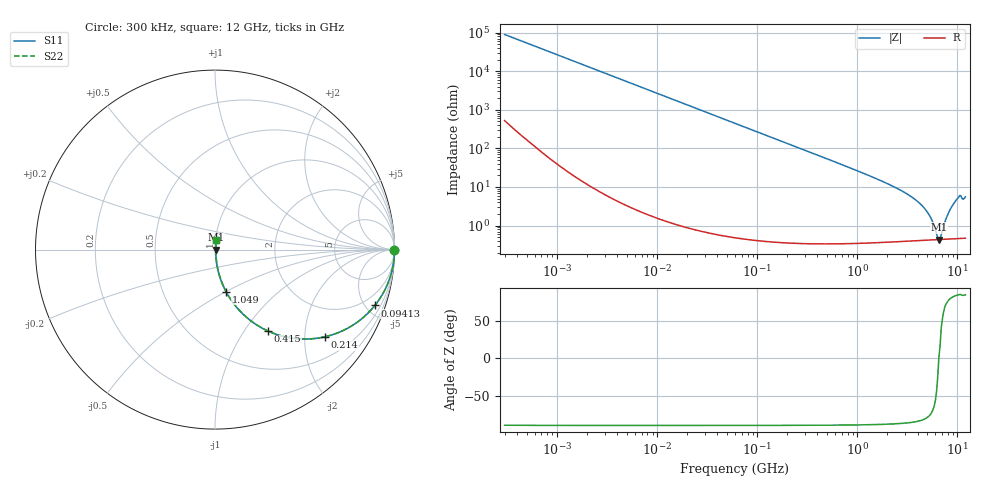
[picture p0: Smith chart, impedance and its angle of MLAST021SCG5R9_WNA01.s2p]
! MLAST021SCG5R9_WNA01  S-PARAMETER MODEL  ( General Type )
! Model Generated by TAIYO YUDEN Corporation (http://www.ty-top.com)
! Version 1.0
! TAIYO YUDEN Control No. 220901
! Copyright(c) 2022 TAIYO YUDEN CO.,LTD. All Rights Reserved.
! Product Description (link to TY-COMPAS)
! https://ds.yuden.co.jp/TYCOMPAS/or/detail?pn=MLAST021SCG5R9CWNA01&u=M
! Products Name : Multilayer Ceramic Capacitors
! Characteristics :
!  Capacitance : 5.9 pF , Rated Voltage : 25V , TCC : CG / C0G
!  Case Size : 0.25 x 0.125 / 0.0098 x 0.0049 [mm/inch] , Thickness : 0.125 / 0.0049 [mm/inch]
!  (Conditions: Temperature = 25 degC , DC Bias Current/Voltage = 0A / 0V)
! External Node Assignments :
!  1  o---| |---o  2
! GND o---------o GND
! Frequency Range : 0.3MHz  -  12000MHz  [ 401 STEP ]
# MHz S RI R 50
! Freq[MHz].  S11 Real  S11 Imag  S21 Real  S21 Imag  S12 Real  S12 Imag  S22 Real  S22 Imag
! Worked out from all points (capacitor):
!   401 points, 300 kHz to 12 GHz, reference 50 ohm
!   read as one part in series: C = 5.9 pF near 316.3 kHz
!   lowest |Z| = 436 mohm at 6.525 GHz (marker M1)
!   series resonance near 6.515 GHz, so ESL is about 100 pH
!   S11 on the Smith chart (normalised r, x): 300 kHz: open; 94.13 MHz: 1.01, -5.73; 214 MHz: 1.01, -2.52; 415 MHz: 1.01, -1.29; 1.049 GHz: 1.01, -0.50; 12 GHz: 1.01, +0.11
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0.3  1 -0.00111  7.74e-06 0.00111  7.74e-06 0.00111  1 -0.00111
1.769972  1 -0.00656  4.92e-05 0.00656  4.92e-05 0.00656  1 -0.00656
10.44266  0.9985 -0.0387  0.00152 0.0387  0.00152 0.0387  0.9985 -0.0387
27.82928  0.9894 -0.1021  0.0106 0.1021  0.0106 0.1021  0.9894 -0.1021
60  0.9526 -0.2119  0.0474 0.2119  0.0474 0.2119  0.9526 -0.2119
94.13233  0.8911 -0.3108  0.1089 0.3108  0.1089 0.3108  0.8911 -0.3108
213.9924  0.6129 -0.4857  0.3871 0.4857  0.3871 0.4857  0.6129 -0.4857
353.9943  0.3666 -0.4797  0.6334 0.4797  0.6334 0.4797  0.3666 -0.4797
414.98  0.2963 -0.454  0.7037 0.454  0.7037 0.454  0.2963 -0.454
651.0506  0.1461 -0.3491  0.8539 0.3491  0.8539 0.3491  0.1461 -0.3491
1048.836  0.0619 -0.2342  0.9381 0.2342  0.9381 0.2342  0.0619 -0.2342
2088.533  0.0168 -0.1135  0.9832 0.1135  0.9832 0.1135  0.0168 -0.1135
3276.641  0.00766 -0.0607  0.9923 0.0607  0.9923 0.0607  0.00766 -0.0607
4502.883  0.00508 -0.0309  0.9949 0.0309  0.9949 0.0309  0.00508 -0.0309
5278.635  0.00451 -0.0173  0.9955 0.0173  0.9955 0.0173  0.00451 -0.0173
6188.031  0.00432 -0.00413  0.9957 0.00413  0.9957 0.00413  0.00432 -0.00413
6524.734  0.00434 0.000122  0.9957 -0.000122  0.9957 -0.000122  0.00434 0.000122
6879.757  0.00438 0.00372  0.9956 -0.00372  0.9956 -0.00372  0.00438 0.00372
8064.993  0.00484 0.0194  0.9952 -0.0194  0.9952 -0.0194  0.00484 0.0194
9207.246  0.00591 0.037  0.9941 -0.037  0.9941 -0.037  0.00591 0.037
10236.47  0.0074 0.0527  0.9926 -0.0527  0.9926 -0.0527  0.0074 0.0527
12000  0.00771 0.0548  0.9923 -0.0548  0.9923 -0.0548  0.00771 0.0548
